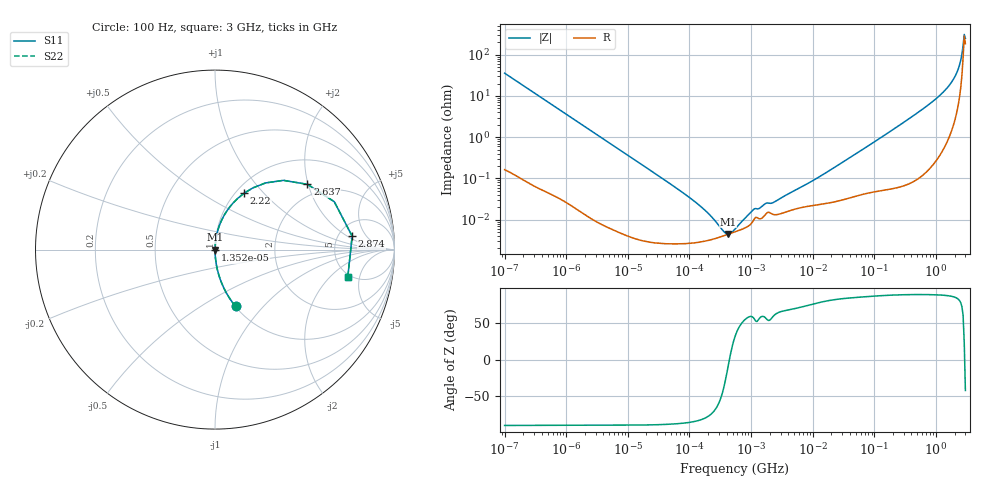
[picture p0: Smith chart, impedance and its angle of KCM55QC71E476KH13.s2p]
!Murata Part Number: KCM55QC71E476KH13
!These Parameters are Measured in Series Mode Connection
!Data Generated on Mar 13, 2026
!  o--ll--o
!Port1  Port2
!  o------o
!Operation Temp=25[degC], DC Bias Voltage=0[V]
!Freq. Start=100[Hz] Stop=3[GHz] 401[Steps]
# Hz S RI R 50
!Freq.(Hz) S11(Real) S11(Imag) S21(Real) S21(Imag) S12(Real) S12(Imag) S22(Real) S22(Imag)
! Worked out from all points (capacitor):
!   401 points, 100 Hz to 3 GHz, reference 50 ohm
!   read as one part in series: C = 44.4 uF near 109 Hz
!   lowest |Z| = 4.47 mohm at 423.1 kHz (marker M1)
!   series resonance near 444.1 kHz, so ESL is about 2.9 nH
!   S11 on the Smith chart (normalised r, x): 100 Hz: 1.00, -0.72; 13.52 kHz: 1.00, -0.01; 2.22 GHz: 1.09, +0.79; 2.637 GHz: 1.64, +1.98; 2.874 GHz: 6.71, +2.44; 3 GHz: 4.72, -3.35
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100  0.1147 -0.3164  0.8853 0.3164  0.8853 0.3164  0.1147 -0.3164
348  0.0111 -0.102  0.9889 0.102  0.9889 0.102  0.0111 -0.102
1788  0.000557 -0.0202  0.9994 0.0202  0.9994 0.0202  0.000557 -0.0202
13520  4.13e-05 -0.00269  1 0.00269  1 0.00269  4.13e-05 -0.00269
31977  2.8e-05 -0.00113  1 0.00113  1 0.00113  2.8e-05 -0.00113
116311  2.73e-05 -0.000289  1 0.000289  1 0.000289  2.73e-05 -0.000289
252400  3.43e-05 -9.3e-05  1 9.3e-05  1 9.3e-05  3.43e-05 -9.3e-05
423062  4.41e-05 -7.3e-06  1 7.3e-06  1 7.3e-06  4.41e-05 -7.3e-06
547723  5.05e-05 3.07e-05  0.9999 -3.07e-05  0.9999 -3.07e-05  5.05e-05 3.07e-05
740304  6e-05 7.64e-05  0.9999 -7.64e-05  0.9999 -7.64e-05  6e-05 7.64e-05
1090550  9.53e-05 0.000147  0.9999 -0.000147  0.9999 -0.000147  9.53e-05 0.000147
1750920  0.00014 0.000207  0.9999 -0.000207  0.9999 -0.000207  0.00014 0.000207
2366551  0.000132 0.000232  0.9999 -0.000232  0.9999 -0.000232  0.000132 0.000232
9794414  0.00022 0.000839  0.9998 -0.000839  0.9998 -0.000839  0.00022 0.000839
1.751444e8  0.000723 0.0134  0.9993 -0.0134  0.9993 -0.0134  0.000723 0.0134
1.06781e9  0.0116 0.0918  0.9884 -0.0918  0.9884 -0.0918  0.0116 0.0918
1.789813e9  0.0567 0.2007  0.9433 -0.2007  0.9433 -0.2007  0.0567 0.2007
2.219584e9  0.1623 0.3143  0.8377 -0.3143  0.8377 -0.3143  0.1623 0.3143
2.419119e9  0.282 0.3715  0.718 -0.3715  0.718 -0.3715  0.282 0.3715
2.636591e9  0.5151 0.3636  0.4849 -0.3636  0.4849 -0.3636  0.5151 0.3636
2.873614e9  0.7642 0.0747  0.2358 -0.0747  0.2358 -0.0747  0.7642 0.0747
3e9  0.7398 -0.1525  0.2602 0.1525  0.2602 0.1525  0.7398 -0.1525
